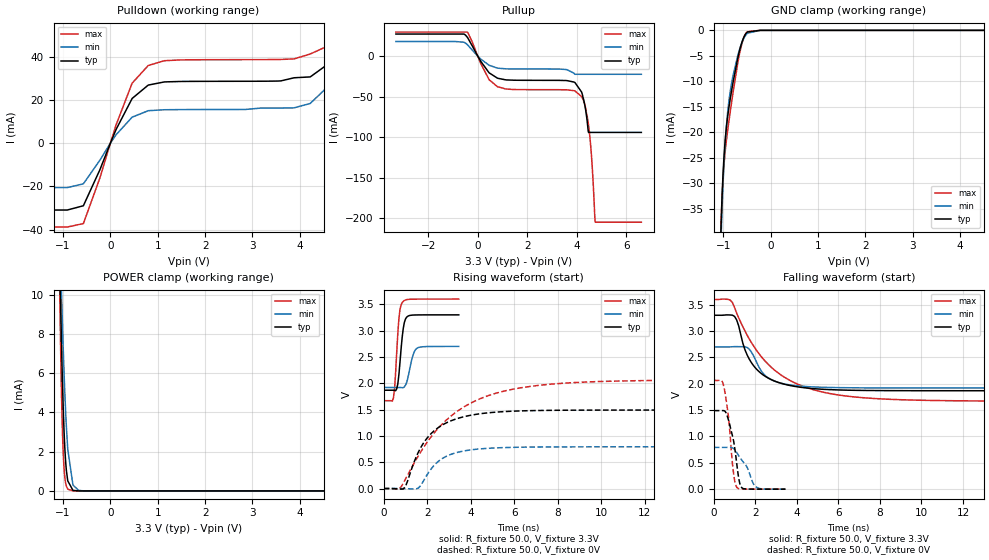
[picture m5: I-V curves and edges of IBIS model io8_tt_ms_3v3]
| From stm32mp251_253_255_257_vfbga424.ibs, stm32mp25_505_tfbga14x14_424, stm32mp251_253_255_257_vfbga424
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[Model]   io8_tt_ms_3v3
Model_type I/O
Polarity   Non-Inverting
Enable   Active-Low
| CAP_THRESHOLD on pad IOTT is "UDTCAPC" :
| Rising=30.0% of vddiov33m   Falling=70.0% of vddiov33m
| C_comp min and max val. don't necessarily correlate with the min and max pvt
| but are the smallest and greatest pad capacitance found.
| var   typ   min   max
C_comp   1.23987pF  995.24944fF  2.17617pF
|C_comp_pullup   730.17000fF  473.44500fF  1.67078pF
|C_comp_pulldown   509.69500fF  521.80444fF  505.38500fF
Vinl = 810.0mV
Vinh = 2.52V
Vmeas = 1.65V   | Reference voltage for timing measurements
Cref  = 50.0pF   | Timing specification test load capacitance value
Rref  = 100.0MOhm   | Timing specification test load resistance value
Vref  = 1.65V   | Timing specification test load voltage
[Model Spec]
| TIME_THRESHOLD on pin ZIV08M is "CMOS" :
| Rising=50.0% of vddv08m   Falling=50.0% of vddv08m
Vinl 1.08570V 868.70000mV 1.21270V
Vinh 1.55630V 1.26330V 1.71030V
| variable   typ   min   max
[Temperature Range] 25.0 125.0 -40.0
| variable   typ   min   max
[Voltage Range] 3.3V 2.7V 3.6V
| variable   typ   min   max
[POWER Clamp Reference] 3.3V 2.7V 3.6V
| variable   typ   min   max
[GND Clamp Reference] 0V 0V 0V
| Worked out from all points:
|   slope of the pulldown table from 0 to 0.495 V, typ, clamps not added: 23.2 ohm
|   slope of the pullup table from 0 to 0.495 V, typ, clamps not added: 23.2 ohm
|   GND clamp passes 1 mA (typ) near -0.55 V on its own axis
|   POWER clamp passes 1 mA (typ) near -0.93 V on its own axis
|   rising waveform, R_fixture 50.0, V_fixture 3.3V: 20-80 % time 195ps typ, 261ps min, 172ps max; typ from 1.87 V to 3.3 V
|   falling waveform, R_fixture 50.0, V_fixture 3.3V: 20-80 % time 1.18ns typ, 882ps min, 2.47ns max; typ from 3.3 V to 1.87 V
|   rising waveform, R_fixture 50.0, V_fixture 0V: 20-80 % time 1.42ns typ, 1.15ns min, 2.83ns max; typ from 0 V to 1.49 V
|   falling waveform, R_fixture 50.0, V_fixture 0V: 20-80 % time 380ps typ, 641ps min, 308ps max; typ from 1.49 V to 0 V
[POWER Clamp]
-3.3V     1.352A     318.4mA    1.997A
-1.07V    12.07mA    13.62mA    10.38mA
-1.06V    10.79mA    12.67mA    8.742mA
-1.05V    9.57mA     11.75mA    7.25mA
-1.03V    7.34mA     9.996mA    4.745mA
-1V       4.587mA    7.593mA    2.212mA
-980mV    3.182mA    6.169mA    1.235mA
-950mV    1.703mA    4.334mA    479uA
-900mV    514.7uA    2.139mA    90.77uA
-790mV    28.73uA    299.9uA    2.711uA
-670mV    1.278uA    27.54uA    387.5nA
6.6V      0A         0A         0A
[GND Clamp]
-3.3V     -3.764A    -3.734A    -3.781A
-1.05V    -39.76mA   -42.44mA   -39.2mA
-1.04V    -36.65mA   -39.24mA   -36.3mA
-1.03V    -33.91mA   -36.36mA   -33.82mA
-1V       -27.43mA   -29.21mA   -28.35mA
-970mV    -22.87mA   -23.78mA   -24.78mA
-920mV    -17.9mA    -17.36mA   -20.6mA
-860mV    -13.88mA   -12.47mA   -16.46mA
-790mV    -10.04mA   -8.727mA   -11.99mA
-650mV    -3.744mA   -3.565mA   -4.327mA
-490mV    -324.2uA   -555.2uA   -259.7uA
6.6V      204.7nA    4.775uA    218.9nA
| variable   typ   min   max
[Pullup Reference] 3.3V 2.7V 3.6V
| variable   typ   min   max
[Pulldown Reference] 0V 0V 0V
[Pullup]
-3.3V     27.2mA     17.98mA    29.6mA
-430mV    23.6mA     14.4mA     29.53mA
460mV     -20.66mA   -11.32mA   -29.13mA
800mV     -27.28mA   -14.86mA   -37.8mA
3.92V     -32.58mA   -22.41mA   -42.95mA
4.21V     -46.24mA   -22.41mA   -50.96mA
4.34V     -63.96mA   -22.41mA   -62.51mA
4.44V     -87.52mA   -22.41mA   -78.87mA
4.47V     -94.08mA   -22.41mA   -85.37mA
4.59V     -94.08mA   -22.41mA   -123.9mA
4.74V     -94.08mA   -22.41mA   -204.6mA
6.6V      -94.08mA   -22.41mA   -204.7mA
[Pulldown]
-3.3V     -30.93mA   -20.55mA   -38.82mA
-570mV    -28.96mA   -18.8mA    -37.2mA
-220mV    -12.23mA   -7.828mA   -16.04mA
120mV     6.335mA    3.893mA    8.43mA
460mV     20.73mA    12.07mA    27.81mA
800mV     26.92mA    15.05mA    35.98mA
3.88V     30.3mA     16.38mA    39.04mA
4.22V     30.7mA     18.4mA     41.31mA
4.56V     36.08mA    25.54mA    44.69mA
4.9V      54.47mA    48.35mA    60.15mA
5.24V     110.5mA    112.9mA    109.4mA
6.6V      684.9mA    689.2mA    638.4mA
[Ramp]
dV/dt_r 894.61079mV/1.41519ns 475.73583mV/1.14947ns 1.23806V/2.82815ns
dV/dt_f 859.29651mV/1.17403ns 467.97371mV/880.95798ps 1.15861V/2.46771ns
R_load = 50.0
| Removed startup time: 0s 0s 0s  .
| Removed end time: 3.45ns.
[Rising Waveform]
R_fixture   = 50.0
V_fixture   = 3.3V
V_fixture_min = 2.7V
V_fixture_max = 3.6V
0s        1.868V     1.92V      1.669V
450ps     1.868V     1.92V      1.722V
550ps     1.859V     1.92V      2.199V
650ps     1.986V     1.92V      2.943V
750ps     2.397V     1.92V      3.403V
850ps     2.87V      1.916V     3.531V
1.05ns    3.252V     2.008V     3.588V
1.3ns     3.294V     2.464V     3.597V
1.5ns     3.298V     2.657V     3.598V
3.45ns    3.3V       2.7V       3.6V
| Removed startup time: 0s 0s 0s  .
| Removed end time: 24.9ns.
[Falling Waveform]
R_fixture   = 50.0
V_fixture   = 3.3V
V_fixture_min = 2.7V
V_fixture_max = 3.6V
0s        3.3V       2.7V       3.6V
700ps     3.307V     2.7V       3.601V
1ns       3.279V     2.705V     3.449V
1.2ns     3.097V     2.704V     3.25V
1.6ns     2.553V     2.69V      2.928V
2.4ns     2.162V     2.185V     2.462V
3.7ns     1.965V     1.976V     2.057V
5.4ns     1.893V     1.932V     1.829V
9.9ns     1.869V     1.92V      1.688V
24.9ns    1.868V     1.92V      1.669V
| Removed startup time: 0s 0s 0s  .
| Removed end time: 24.9ns.
[Rising Waveform]
R_fixture   = 50.0
V_fixture   = 0V
V_fixture_min = 0V
V_fixture_max = 0V
0s        423.1nV    2.43uV     511.3nV
700ps     -7.245mV   -113.8uV   -9.586mV
900ps     -8.876mV   -1.731mV   100.8mV
1.5ns     606.7mV    -5.868mV   555.7mV
1.8ns     845mV      124.4mV    759.7mV
2.7ns     1.208V     571.8mV    1.23V
4.1ns     1.4V       739.2mV    1.644V
5.9ns     1.469V     781.9mV    1.884V
10.9ns    1.491V     792.7mV    2.043V
24.9ns    1.491V     792.9mV    2.063V
| Removed startup time: 0s 0s 0s  .
| Removed end time: 3.45ns.
[Falling Waveform]
R_fixture   = 50.0
V_fixture   = 0V
V_fixture_min = 0V
V_fixture_max = 0V
0s        1.491V     792.9mV    2.064V
400ps     1.491V     792.9mV    2.049V
500ps     1.489V     792.9mV    1.919V
700ps     1.324V     793mV      1.402V
950ps     925mV      772.9mV    307.9mV
1.1ns     501.8mV    698.9mV    38.44mV
1.25ns    111.7mV    605.8mV    6.944mV
1.4ns     13.92mV    524.2mV    2.959mV
2.05ns    826.7uV    38.96mV    891.4uV
3.45ns    218.6uV    231.2uV    268uV
